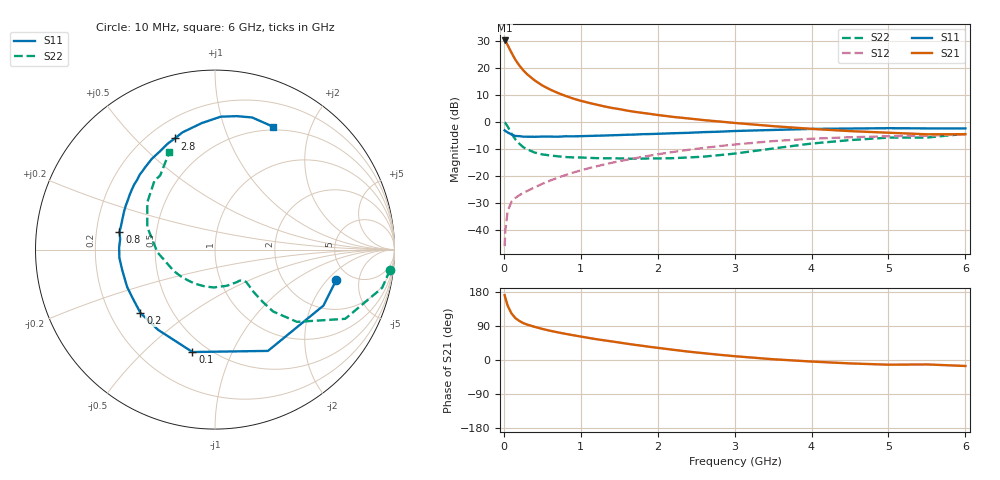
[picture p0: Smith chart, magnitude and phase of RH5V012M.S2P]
! SIEMENS Small Signal Semiconductors
! BFR106
! Si NPN RF Bipolar Junction Transistor in SOT23
! VCE = 5 V  IC = 12 mA
! Common Emitter S-Parameters:  August  1996
# GHz  S  MA  R  50
!  f  S11  S21  S12  S22
! GHz  MAG  ANG  MAG  ANG  MAG  ANG  MAG  ANG
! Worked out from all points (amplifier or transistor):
!   36 points, 10 MHz to 6 GHz, reference 50 ohm
!   highest |S21| = 30.2 dB at 10 MHz (marker M1)
!   |S21| within 3 dB of that: start of sweep to 72.63 MHz
!   unconditionally stable (mu >= 1): 456.1 MHz to 2.024 GHz; 5.368 GHz to end of sweep
!   at 250 MHz: K = 0.76, MSG = 22.7 dB, |S12| = -26.3 dB
!   at 1.4 GHz: K = 1.08, MAG = 8.4 dB, |S12| = -15.2 dB
!   at 6 GHz: K = 1.00, MAG = -0.3 dB, |S12| = -4.6 dB
!   S11 on the Smith chart (normalised r, x): 10 MHz: 3.86, -2.52; 100 MHz: 0.41, -0.72; 200 MHz: 0.33, -0.33; 800 MHz: 0.30, +0.08; 2.8 GHz: 0.30, +0.66; 6 GHz: 0.46, +1.48
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0.01  0.6965 -14.0  32.19 171.0  0.005 86.4  0.9815 -6.6
0.02  0.6801 -27.3  31.27 163.6  0.0099 78.6  0.9554 -12.9
0.05  0.6369 -62.4  26.41 143.3  0.0224 63.8  0.8215 -28.0
0.1  0.5843 -102.4  19.06 122.9  0.0335 52.3  0.609 -41.4
0.15  0.5481 -125.4  14.13 110.5  0.0391 48.6  0.473 -46.8
0.2  0.5451 -139.6  11.16 103.3  0.0438 49.6  0.3964 -47.6
0.25  0.5325 -149.8  9.09 97.6  0.0484 50.4  0.342 -47.7
0.3  0.5319 -157.0  7.684 93.7  0.0522 52.7  0.3117 -47.6
0.4  0.5293 -167.3  5.871 87.5  0.0613 55.5  0.2709 -46.5
0.5  0.5347 -175.0  4.724 82.0  0.0713 58.4  0.2502 -46.1
0.6  0.5344 178.8  3.983 77.3  0.0817 60.6  0.2393 -46.9
0.8  0.5412 169.5  3.031 69.1  0.1035 62.5  0.2236 -50.4
0.9  0.5402 165.5  2.709 65.4  0.1151 63.1  0.2201 -52.3
1.1  0.5496 157.1  2.262 58.4  0.1384 63.6  0.2163 -58.9
1.3  0.5583 150.5  1.944 52.0  0.1623 62.9  0.212 -65.4
1.6  0.578 141.2  1.62 43.0  0.1994 61.1  0.2092 -77.9
2.2  0.6162 124.8  1.237 27.0  0.2776 55.0  0.213 -107.3
2.8  0.6584 109.9  1.017 13.8  0.3557 46.8  0.2423 -142.4
3.5  0.709 95.9  0.834 2.0  0.4407 35.7  0.3216 -177.4
4.5  0.7534 80.7  0.675 -9.0  0.5195 18.7  0.4599 145.1
5.5  0.7577 68.6  0.589 -11.7  0.555 7.2  0.5133 126.5
6  0.7572 64.8  0.592 -15.8  0.5881 -0.6  0.6005 115.1
